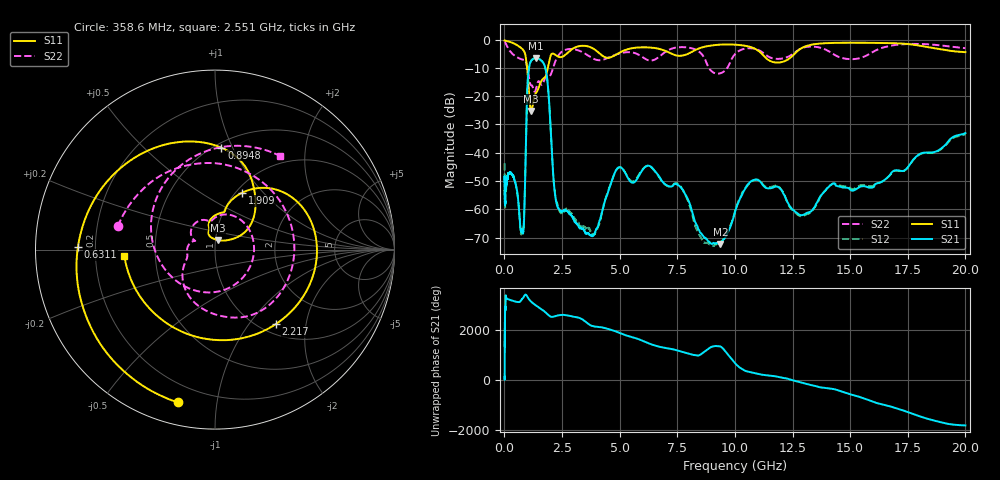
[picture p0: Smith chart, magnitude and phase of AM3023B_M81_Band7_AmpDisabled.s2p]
!Agilent Technologies,E8364B,MY43040894,A.07.50.67
!Agilent E8364B: A.07.50.67
!Date: Tuesday, October 27, 2020 10:40:16
!Correction: S11(Full 2 Port(1,2))
!S21(Full 2 Port(1,2))
!S12(Full 2 Port(1,2))
!S22(Full 2 Port(1,2))
!S2P File: Measurements: S11, S21, S12, S22:Log Frequency Sweep
# Hz S  dB  R 50
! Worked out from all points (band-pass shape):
!   3201 points, 10 MHz to 20 GHz, reference 50 ohm
!   highest |S21| = -6.59 dB at 1.362 GHz (marker M1); lowest = -72.3 dB at 9.375 GHz (marker M2)
!   |S21| within 3 dB of the highest: 1.076 GHz to 1.763 GHz (686.7 MHz wide, 48.4 % of centre)
!   lowest |S11| = -25.2 dB at 1.159 GHz (marker M3), VSWR 1.12, Z = 51.1 + j5.45 ohm
!   |S11| at or under -10 dB: 986.6 MHz to 1.885 GHz (898.6 MHz wide, 62.6 % of centre)
!   |S22| runs from -18.4 to -0.6 dB; largest |S21 - S12| = 0.0092
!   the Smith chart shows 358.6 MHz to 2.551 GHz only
!   S11 on the Smith chart (normalised r, x): 358.6 MHz: 0.11, -0.78; 631.1 MHz: 0.13, +0.01; 894.8 MHz: 0.54, +0.91; 1.909 GHz: 1.07, +0.77; 2.217 GHz: 1.17, -1.37; 2.551 GHz: 0.33, -0.03
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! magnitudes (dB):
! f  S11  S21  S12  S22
! 10 MHz  -0.3  -50.3  -43.7  -0.7
! 35.55 MHz  -0.4  -57.7  -57.7  -0.9
! 126.1 MHz  -0.5  -49.1  -48.2  -2.5
! 358.6 MHz  -1.1  -48.0  -48.1  -5.1
! 447.2 MHz  -1.5  -49.9  -49.6  -5.7
! 631.1 MHz  -2.3  -59.9  -59.5  -6.6
! 813.7 MHz  -3.6  -68.3  -67.0  -7.1
! 894.8 MHz  -4.9  -51.9  -52.1  -7.3
! 1.005 GHz  -11.6  -15.9  -15.9  -10.3
! 1.159 GHz  -25.2  -7.5  -7.5  -16.1
! 1.362 GHz  -18.9  -6.6  -6.6  -17.7
! 1.59 GHz  -14.8  -7.3  -7.3  -15.8
! 1.909 GHz  -9.1  -18.4  -18.4  -13.3
! 2.217 GHz  -5.4  -56.0  -55.8  -7.5
! 2.551 GHz  -5.9  -60.5  -61.1  -3.9
! 3.802 GHz  -2.9  -69.4  -68.8  -6.5
! 4.89 GHz  -5.1  -45.6  -45.7  -5.1
! 5.639 GHz  -2.9  -50.4  -50.0  -4.7
! 9.375 GHz  -1.8  -72.3  -71.9  -11.9
! 10.73 GHz  -2.7  -49.9  -50.1  -3.1
! 13.01 GHz  -2.5  -61.8  -62.2  -2.7
! 20 GHz  -4.4  -33.0  -33.4  -3.0
